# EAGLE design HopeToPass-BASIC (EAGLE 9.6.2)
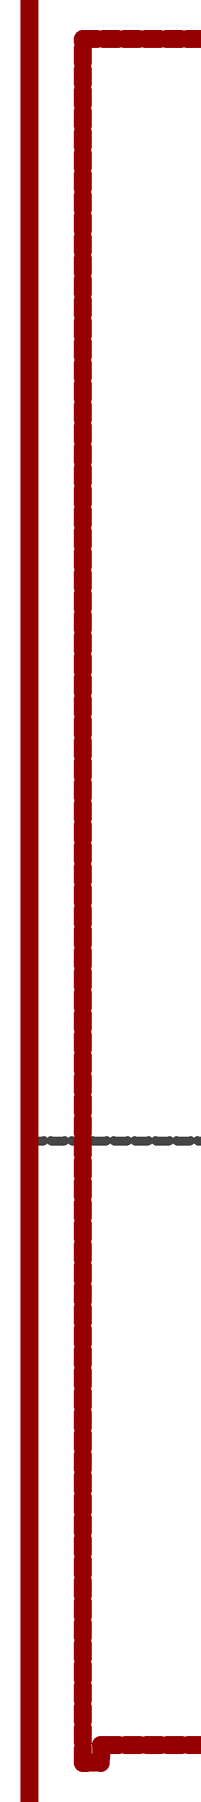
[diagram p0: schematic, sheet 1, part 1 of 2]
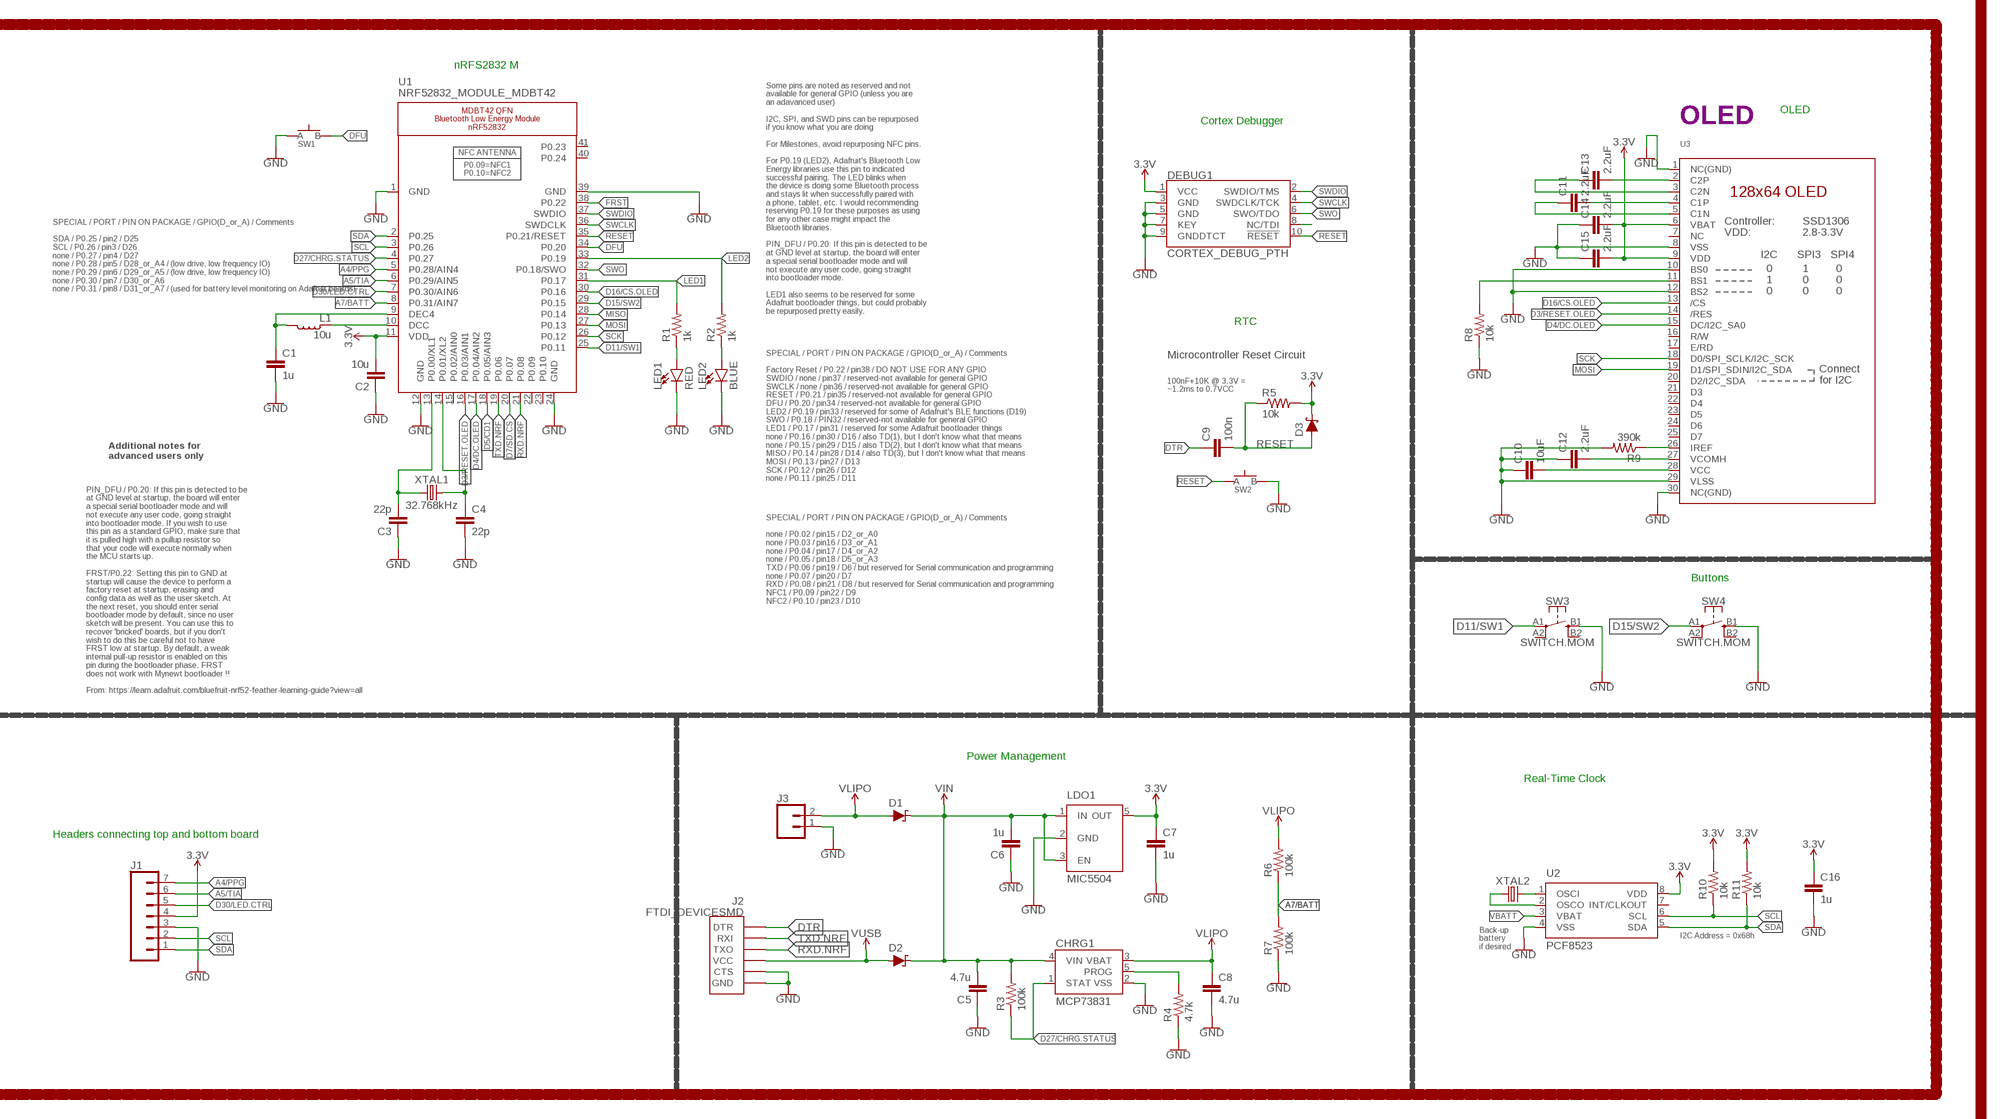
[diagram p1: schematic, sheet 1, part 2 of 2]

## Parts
C1  1u  CAPACITOR0603  [C0603]
C2  10u  CAPACITOR0805  [C0805]
C3  22p  CAPACITOR0603  [C0603]
C4  22p  CAPACITOR0603  [C0603]
C5  4.7u  CAPACITOR0603  [C0603]
C6  1u  CAPACITOR0603  [C0603]
C7  1u  CAPACITOR0603  [C0603]
C8  4.7u  CAPACITOR0603  [C0603]
C9  100n  CAPACITOR0603  [C0603]
C10  10uF  CAPACITOR0603  [C0603]
C11  2.2uF  CAPACITOR0603  [C0603]
C12  2.2uF  CAPACITOR0603  [C0603]
C13  2.2uF  CAPACITOR0603  [C0603]
C14  2.2uF  CAPACITOR0603  [C0603]
C15  2.2uF  CAPACITOR0603  [C0603]
C16  1u  CAPACITOR0603  [C0603]
CHRG1  MCP73831  [SOT23-5]
D1  SCHOTTKY-USC  [USC]
D2  SCHOTTKY-USC  [USC]
D3  SCHOTTKY-USC  [USC]
DEBUG1  CORTEX_DEBUG_PTH  [2X5-PTH-1.27MM]
J1  CONN_07-1.27MM  [1X07_1.27MM]
J2  FTDI_DEVICESMD  [FTDI-SMD]
J3  CONN_02  [1X02]
L1  10u  INDUCTOR0603  [L0603]
LDO1  MIC5504  [SOT23-5]
LED1  RED  LED0603  [LED-0603]
LED2  BLUE  LED0603  [LED-0603]
R1  1k  RESISTOR0603  [R0603]
R2  1k  RESISTOR0603  [R0603]
R3  100k  RESISTOR0603  [R0603]
R4  4.7k  RESISTOR0603  [R0603]
R5  10k  RESISTOR0603  [R0603]
R6  100k  RESISTOR0603  [R0603]
R7  100k  RESISTOR0603  [R0603]
R8  10k  RESISTOR0603  [R0603]
R9  390k  RESISTOR0603  [R0603]
R10  10k  RESISTOR0603  [R0603]
R11  10k  RESISTOR0603  [R0603]
SW1  SPST-PTS830GG140-COPY.1-3  [BUTTON-GULLWING]
SW2  SPST-PTS830GG140-COPY.1-3  [BUTTON-GULLWING]
SW3  SWITCH.MOM  [TACTILE_SWITCH_SMD_6.2MM_TALL]
SW4  SWITCH.MOM  [TACTILE_SWITCH_SMD_6.2MM_TALL]
U1  NRF52832_MODULE_MDBT42  [BLE_MODULE_RAYTAC_MDBT42]
U2  PCF8523  [SO8]
U3  DISP_OLED_UG-2864HSWEG01-NO-WRAPAROUND  [UG-2864HSWEG01_0.96IN_NO-WRAPAROUND]
XTAL1  32.768kHz  CRYSTALECS-.327-12.5-12-C-TR  [2-SMD.NOLEAD.2.0MMTO1.2MM]
XTAL2  32.7680kHz  CRYSTALECS-.327-12.5-12-C-TR  [2-SMD.NOLEAD.2.0MMTO1.2MM]

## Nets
3.3V: C2.2 C7.1 C14.2 C15.2 C16.1 D3.-(C) DEBUG1.1(VCC) J1.4 LDO1.5(OUT) R5.2 R10.2 R11.2 U1.11(VDD) U2.8(VDD) U3.6(VBAT) U3.9(VDD)
A4/PPG: J1.7 U1.5(P0.28/AIN4)
A5/TIA: J1.6 U1.6(P0.29/AIN5)
A7/BATT: R6.1 R7.2 U1.8(P0.31/AIN7)
D3/RESET.OLED: U1.16(P0.03/AIN1) U3.14(/RES)
D4/DC.OLED: U1.17(P0.04/AIN2) U3.15(DC/I2C_SA0)
D5/CD1: U1.18(P0.05/AIN3)
D7/SD.CS: U1.20(P0.07)
D11/SW1: SW3.A1 U1.25(P0.11)
D15/SW2: SW4.A1 U1.29(P0.15)
D16/CS.OLED: U1.30(P0.16) U3.13(/CS)
D27/CHRG.STATUS: CHRG1.1(STAT) R3.1 U1.4(P0.27)
D30/LED.CTRL: J1.5 U1.7(P0.30/AIN6)
DFU: SW1.3(B) U1.34(P0.20)
DTR: C9.1 J2.DTR
FRST: U1.38(P0.22)
GND: C1.2 C2.1 C3.1 C4.2 C5.1 C6.1 C7.2 C8.2 C10.1 C12.1 C14.1 C15.1 C16.2 CHRG1.2(VSS) DEBUG1.3(GND) DEBUG1.5(GND) DEBUG1.7(KEY) DEBUG1.9(GNDDTCT) J1.3 J2.CTS J2.GND J3.1 LDO1.2(GND) LED1.C LED2.C R4.1 R7.1 R8.1 R9.2 SW1.1(A) SW2.3(B) SW3.B1 SW4.B1 U1.1(GND) U1.12(GND) U1.24(GND) U1.39(GND) U2.4(VSS) U3.1(NC(GND)) U3.8(VSS) U3.10(BS0) U3.12(BS2) U3.29(VLSS) U3.30(NC(GND))
LED1: R1.2 U1.31(P0.17)
LED2: R2.2 U1.33(P0.19)
MISO: U1.28(P0.14)
MOSI: U1.27(P0.13) U3.19(D1/SPI_SDIN/I2C_SDA)
N$1: R8.2 U3.11(BS1)
N$2: R9.1 U3.26(IREF)
N$3: C13.2 U3.2(C2P)
N$4: C3.2 U1.13(P0.00/XL1) XTAL1.P$1
N$5: C13.1 U3.3(C2N)
N$6: C4.1 U1.14(P0.01/XL2) XTAL1.P$2
N$7: C11.2 U3.4(C1P)
N$8: C11.1 U3.5(C1N)
N$9: LED1.A R1.1
N$10: LED2.A R2.1
N$11: L1.1 U1.10(DCC)
N$12: C1.1 L1.2 U1.9(DEC4)
N$13: C10.2 U3.28(VCC)
N$14: DEBUG1.8(NC/TDI)
N$15: C12.2 U3.27(VCOMH)
N$17: CHRG1.5(PROG) R4.2
N$21: U2.2(OSCO) XTAL2.P$1
N$22: U2.1(OSCI) XTAL2.P$2
RESET: C9.2 D3.+(A) DEBUG1.10(!RESET) R5.1 SW2.1(A) U1.35(P0.21/RESET)
RXD.NRF: J2.TXO U1.21(P0.08)
SCK: U1.26(P0.12) U3.18(D0/SPI_SCLK/I2C_SCK)
SCL: J1.2 R10.1 U1.3(P0.26) U2.6(SCL)
SDA: J1.1 R11.1 U1.2(P0.25) U2.5(SDA)
SWCLK: DEBUG1.4(SWDCLK/TCK) U1.36(SWDCLK)
SWDIO: DEBUG1.2(SWDIO/TMS) U1.37(SWDIO)
SWO: DEBUG1.6(SWO/TDO) U1.32(P0.18/SWO)
TXD.NRF: J2.RXI U1.19(P0.06)
V_USB: D2.+(A) J2.VCC ; supply symbol labelled VUSB
VBATT: U2.3(VBAT)
VIN: C5.2 C6.2 CHRG1.4(VIN) D1.-(C) D2.-(C) LDO1.1(IN) LDO1.3(EN) R3.2
VLIPO: C8.1 CHRG1.3(VBAT) D1.+(A) J3.2 R6.2
Unconnected: SW3.A2 SW3.B2 SW4.A2 SW4.B2 U1.15(P0.02/AIN0) U1.22(P0.09) U1.23(P0.10) U1.40(P0.24) U1.41(P0.23) U2.7(INT/CLKOUT) U3.7(NC) U3.16(R/W) U3.17(E/RD) U3.20(D2/I2C_SDA) U3.21(D3) U3.22(D4) U3.23(D5) U3.24(D6) U3.25(D7)

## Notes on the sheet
- nRFS2832 M
- OLED
- Cortex Debugger | OLED
- SPECIAL / PORT / PIN ON PACKAGE / GPIO(D_or_A) / Comments
  
  SDA / P0.25 / pin2 / D25
  SCL / P0.26 / pin3 / D26
  none / P0.27 / pin4 / D27
  none / P0.28 / pin5 / D28_or_A4 / (low drive, low frequency IO)
  none / P0.29 / pin6 / D29_or_A5 / (low drive, low frequency IO)
  none / P0.30 / pin7 / D30_or_A6
  none / P0.31 / pin8 / D31_or_A7 / (used for battery level monitoring on Adafruit boards)
- Some pins are noted as reserved and not
  available for general GPIO (unless you are
  an adavanced user)
  
  I2C, SPI, and SWD pins can be repurposed
  if you know what you are doing
  
  For Milestones, avoid repurposing NFC pins.
  
  For P0.19 (LED2), Adafruit's Bluetooth Low
  Energy libraries use this pin to indicated
  successful pairing. The LED blinks when
  the device is doing some Bluetooth process
  and stays lit when successfully paired with
  a phone, tablet, etc. I would recommending
  reserving P0.19 for these purposes as using
  for any other case might impact the
  Bluetooth libraries.
  
  PIN_DFU / P0.20: If this pin is detected to be
  at GND level at startup, the board will enter
  a special serial bootloader mode and will
  not execute any user code, going straight
  into bootloader mode.
  
  LED1 also seems to be reserved for some
  Adafruit bootloader things, but could probably
  be repurposed pretty easily.
- RTC
- Microcontroller Reset Circuit
- 100nF+10K @ 3.3V =
  ~1.2ms to 0.7VCC
- Additional notes for
  advanced users only
- SPECIAL / PORT / PIN ON PACKAGE / GPIO(D_or_A) / Comments
  
  Factory Reset / P0.22 / pin38 / DO NOT USE FOR ANY GPIO
  SWDIO / none / pin37 / reserved-not available for general GPIO
  SWCLK / none / pin36 / reserved-not available for general GPIO
  RESET / P0.21 / pin35 / reserved-not available for general GPIO
  DFU / P0.20 / pin34 / reserved-not available for general GPIO
  LED2 / P0.19 / pin33 / reserved for some of Adafruit's BLE functions (D19)
  SWO / P0.18 / PIN32 / reserved-not available for general GPIO
  LED1 / P0.17 / pin31 / reserved for some Adafruit bootloader things
  none / P0.16 / pin30 / D16 / also TD(1), but I don't know what that means
  none / P0.15 / pin29 / D15 / also TD(2), but I don't know what that means
  MISO / P0.14 / pin28 / D14 / also TD(3), but I don't know what that means
  MOSI / P0.13 / pin27 / D13
  SCK / P0.12 / pin26 / D12
  none / P0.11 / pin25 / D11
- Buttons
- SPECIAL / PORT / PIN ON PACKAGE / GPIO(D_or_A) / Comments
  
  none / P0.02 / pin15 / D2_or_A0
  none / P0.03 / pin16 / D3_or_A1
  none / P0.04 / pin17 / D4_or_A2
  none / P0.05 / pin18 / D5_or_A3
  TXD / P0.06 / pin19 / D6 / but reserved for Serial communication and programming
  none / P0.07 / pin20 / D7
  RXD / P0.08 / pin21 / D8 / but reserved for Serial communication and programming
  NFC1 / P0.09 / pin22 / D9
  NFC2 / P0.10 / pin23 / D10
- PIN_DFU / P0.20: If this pin is detected to be
  at GND level at startup, the board will enter
  a special serial bootloader mode and will
  not execute any user code, going straight
  into bootloader mode. If you wish to use
  this pin as a standard GPIO, make sure that
  it is pulled high with a pullup resistor so
  that your code will execute normally when
  the MCU starts up.
  
  FRST/P0.22: Setting this pin to GND at
  startup will cause the device to perform a
  factory reset at startup, erasing and
  config data as well as the user sketch. At
  the next reset, you should enter serial
  bootloader mode by default, since no user
  sketch will be present. You can use this to
  recover 'bricked' boards, but if you don't
  wish to do this be careful not to have
  FRST low at startup. By default, a weak
  internal pull-up resistor is enabled on this
  pin during the bootloader phase. FRST
  does not work with Mynewt bootloader !!
  
  From: https://learn.adafruit.com/bluefruit-nrf52-feather-learning-guide?view=all
- Power Management
- Real-Time Clock
- Headers connecting top and bottom board
- I2C Address = 0x68h
- Back-up
  battery
  if desired

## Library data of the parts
C1-C16 = LinnesLab-Passives:CAPACITOR
CHRG1 = LinnesLab-Power:MCP73831: MCP73831T Li-Ion, Li-Pol Controller Miniature single cell, fully integrated Li-Ion, Li-polymer charge management controller Datasheet SparkFun Products: SparkFun ESP32 Thing SparkFun 9DoF Razor IMU M0; PROD_ID: IC-09995
D1-D3 = LinnesLab-DiscreteSemi:SCHOTTKY: Schottky diode
DEBUG1 = LinnesLab-Connectors:CORTEX_DEBUG: Cortex Debug Connector - 10 pin Supports JTAG debug, Serial Wire debug, and Serial Wire Viewer. PTH and SMD connector options available. General Connector Information Products: PTH Connector -via Digi-Key SparkFun PSoc SparkFun T
J1 = LinnesLab-Connectors:CONN_07: Multi connection point. Often used as Generic Header-pin footprint for 0.1 inch spaced/style header connections On any of the 0.1 inch spaced packages, you can populate with these: Break Away Headers - Straight (PRT-00116) Break Away Male Headers - Right Angle (PRT-00553) Female Headers (PRT-00115)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
J2 = LinnesLab-Connectors:FTDI_DEVICE
J3 = LinnesLab-Connectors:CONN_02: Multi connection point. Often used as Generic Header-pin footprint for 0.1 inch spaced/style header connections
L1 = LinnesLab-Passives:INDUCTOR
LDO1 = LinnesLab-Power:MIC5504: MIC5504 Voltage Regulator Output Voltages: 1.0V to 3.3V Input Voltages: 2.5V to 5.5V Link to Datasheet http://ww1.microchip.com/downloads/en/DeviceDoc/MIC550X.pdf
LED1 LED2 = LinnesLab-LED:LED: LED (Generic)
R1-R11 = LinnesLab-Passives:RESISTOR
SW1 SW2 = LinnesLab-Switches:SPST-PTS830GG140-COPY
SW3 SW4 = LinnesLab-Switches:SWITCH.MOM: PTS645SM43SMTR92 LFS
U1 = LinnesLab-Microcontrollers:NRF52832_MODULE_MDBT42: MDBT42 - BLE Module (nRF52832 QFN) VDD: 1.7-3.6V
U2 = LinnesLab-Clocks:PCF8523; DIGIKEY: 568-5306-1-ND; I2C_ADDRESS: 0x68h; MFN: PCF8523T/1,118; MFN_MANUFACTURER: NXP USA Inc.
U3 = LinnesLab-Displays:DISP_OLED_UG-2864HSWEG01: UG-2864HSWEG01 OLED display Both 1.3" and 0.96" models share the same FPC tab footprint, only the screen dimensions vary.
XTAL1 XTAL2 = LinnesLab-Clocks:CRYSTAL; DIGIKEY: XC2288CT-ND; FREQ: 32.7680KHZ; LOAD_CAP: 12.5pF

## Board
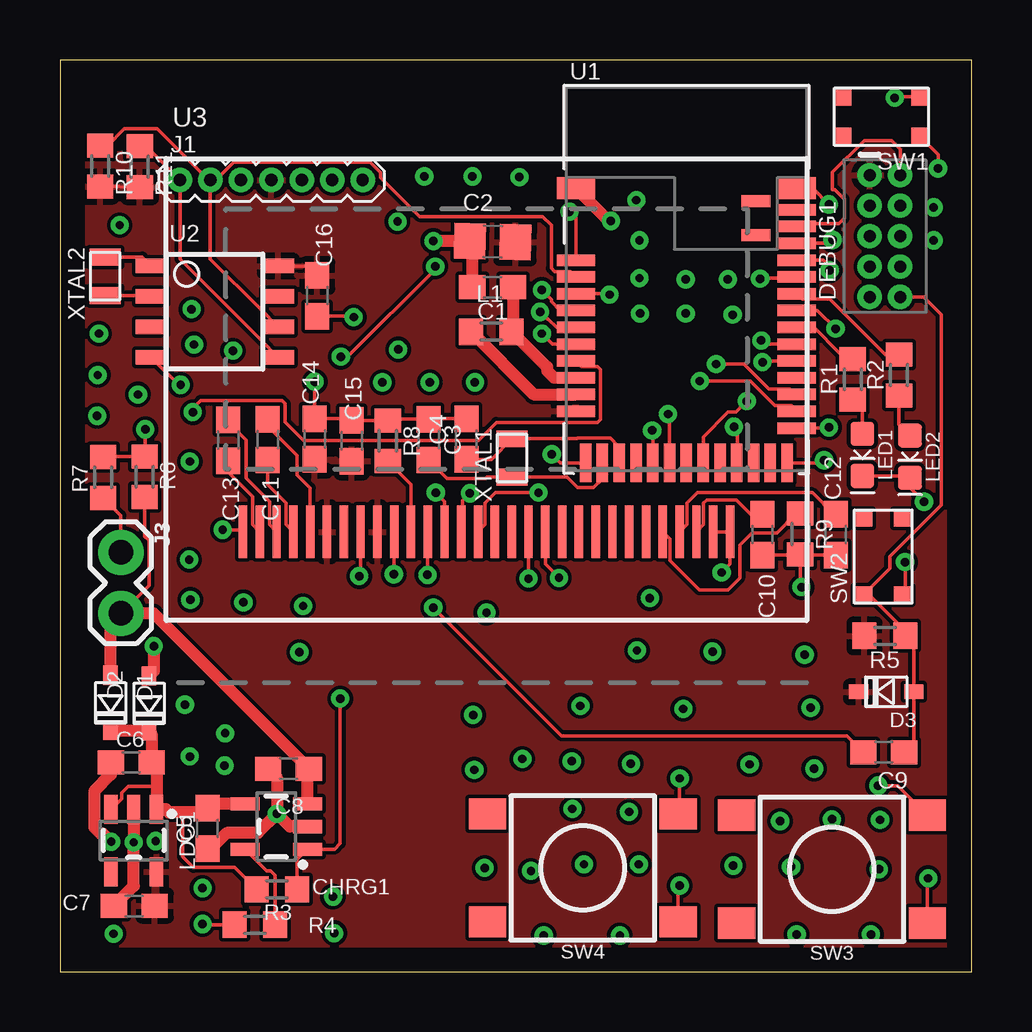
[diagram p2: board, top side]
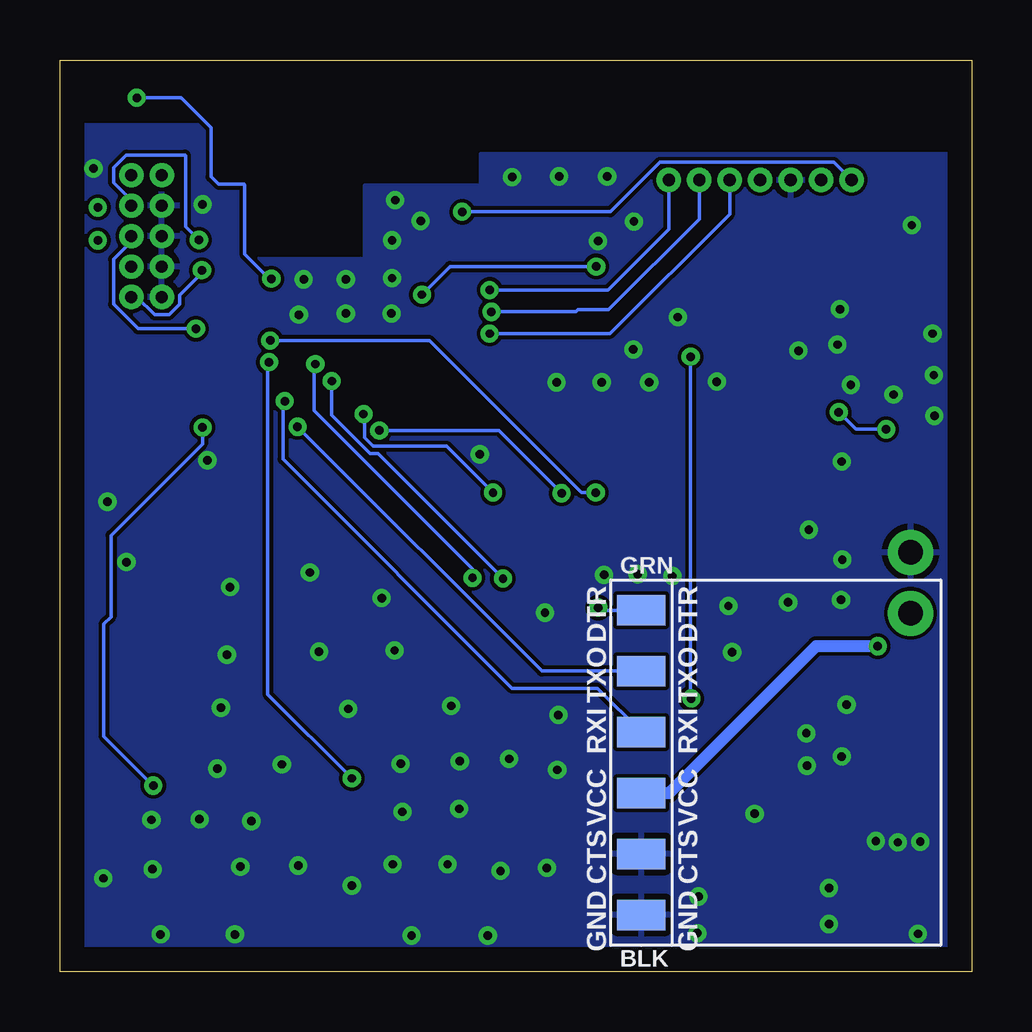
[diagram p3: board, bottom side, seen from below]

Size 38 x 38 mm. Coordinates in mm from the lower left corner, seen from the top.
Outline: 0,0 38,0 38,38 0,38 0,0
Copper layers (1*16): Top 0.035mm / dielectric 1.5mm / Bottom 0.035mm
Design rules "default": minimum track width 6mil, minimum drill 0.35mm, track to track 6mil, track to pad 6mil, pad to pad 6mil, via to via 6mil, smd to smd 6mil, copper to edge 40mil, drill to drill 6mil, minimum pad ring 10mil, minimum via ring 8mil, stop-mask expansion 4mil, vias tented up to drill 0mil, thermal gap 10mil

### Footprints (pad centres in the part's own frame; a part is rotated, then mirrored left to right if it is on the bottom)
C0603 = smd 1.1 x 1: 1 -0.85,0; 2 0.85,0
C0805 = smd 1.3 x 1.5: 1 -0.95,0; 2 0.95,0
SOT23-5 = smd 0.55 x 1.2: 1 -0.95,-1.3; 2 0,-1.3; 3 0.95,-1.3; 4 0.95,1.3; 5 -0.95,1.3
USC = smd 0.8 x 0.6: + -1.15,0; - 1.15,0
2X5-PTH-1.27MM = drill 0.508 pad 1: 1 -2.54,-0.635; 2 -2.54,0.635; 3 -1.27,-0.635; 4 -1.27,0.635; 5 0,-0.635; 6 0,0.635; 7 1.27,-0.635; 8 1.27,0.635; 9 2.54,-0.635; 10 2.54,0.635
1X07_1.27MM = drill 0.508 pad 1: 1 0,0; 2 1.27,0; 3 2.54,0; 4 3.81,0; 5 5.08,0; 6 6.35,0; 7 7.62,0
FTDI-SMD = smd 1.27 x 2.03: CTS 3.81,0; DTR -6.35,0; GND 6.35,0; RXI -1.27,0; TXO -3.81,0; VCC 1.27,0
1X02 = drill 1.016 pad 1.88: 1 0,0; 2 2.54,0
L0603 = smd 1 x 1.1: 1 -0.85,0; 2 0.85,0
LED-0603 = smd 1 x 1: A -0.877,0; C 0.877,0
R0603 = smd 1 x 1.1: 1 -0.85,0; 2 0.85,0
BUTTON-GULLWING = smd 0.7 x 0.75: 1 -1.6,0.825; 2 1.6,0.825; 3 -1.6,-0.825; 4 1.6,-0.825
TACTILE_SWITCH_SMD_6.2MM_TALL = smd 1.55 x 1.3: A1 -3.975,-2.25; A2 3.975,-2.25; B1 -3.975,2.25; B2 3.975,2.25
BLE_MODULE_RAYTAC_MDBT42 = smd 1.6 x 0.9: 1 -4.6,3.8; 39 4.6,3.8 | smd 1.6 x 0.48: 2 -4.6,0.8; 3 -4.6,0.1; 4 -4.6,-0.6; 5 -4.6,-1.3; 6 -4.6,-2; 7 -4.6,-2.7; 8 -4.6,-3.4; 9 -4.6,-4.1; 10 -4.6,-4.8; 11 -4.6,-5.5; 25 4.6,-6.2; 26 4.6,-5.5; 27 4.6,-4.8; 28 4.6,-4.1; 29 4.6,-3.4; 30 4.6,-2.7; 31 4.6,-2; 32 4.6,-1.3; 33 4.6,-0.6; 34 4.6,0.1; 35 4.6,0.8; 36 4.6,1.5; 37 4.6,2.2; 38 4.6,2.9 | smd 0.48 x 1.6: 12 -4.2,-7.65; 13 -3.5,-7.65; 14 -2.8,-7.65; 15 -2.1,-7.65; 16 -1.4,-7.65; 17 -0.7,-7.65; 18 0,-7.65; 19 0.7,-7.65; 20 1.4,-7.65; 21 2.1,-7.65; 22 2.8,-7.65; 23 3.5,-7.65; 24 4.2,-7.65 | smd 1.2 x 0.5: 40 2.9,3.25; 41 2.9,1.85
SO8 = smd 1.3 x 0.6: 1 -2.65,1.905; 2 -2.65,0.635; 3 -2.65,-0.635; 4 -2.65,-1.905; 5 2.65,-1.905; 6 2.65,-0.635; 7 2.65,0.635; 8 2.65,1.905
UG-2864HSWEG01_0.96IN_NO-WRAPAROUND = smd 0.35 x 2.2: 1 -10.15,-1.2; 2 -9.45,-1.2; 3 -8.75,-1.2; 4 -8.05,-1.2; 5 -7.35,-1.2; 6 -6.65,-1.2; 7 -5.95,-1.2; 8 -5.25,-1.2; 9 -4.55,-1.2; 10 -3.85,-1.2; 11 -3.15,-1.2; 12 -2.45,-1.2; 13 -1.75,-1.2; 14 -1.05,-1.2; 15 -0.35,-1.2; 16 0.35,-1.2; 17 1.05,-1.2; 18 1.75,-1.2; 19 2.45,-1.2; 20 3.15,-1.2; 21 3.85,-1.2; 22 4.55,-1.2; 23 5.25,-1.2; 24 5.95,-1.2; 25 6.65,-1.2; 26 7.35,-1.2; 27 8.05,-1.2; 28 8.75,-1.2; 29 9.45,-1.2; 30 10.15,-1.2
2-SMD.NOLEAD.2.0MMTO1.2MM = smd 0.7 x 1.3: P$1 -0.8,0; P$2 0.8,0

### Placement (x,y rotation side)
C1  18.03,28.52 180 top
C2  18.03,30.43 358.7 top
C3  15.37,22.17 270 top
C4  16.94,22.2 90 top
C5  6.15,5.97 90 top
C6  2.97,8.71 0 top
C7  3.1,2.74 180 top
C8  9.53,8.46 180 top
C9  34.34,9.14 0 top
C10  29.29,18.21 90 top
C11  8.66,22.17 270 top
C12  32.33,18.21 90 top
C13  7.01,22.15 270 top
C14  10.62,22.2 270 top
C15  12.17,22.12 270 top
C16  10.72,28.17 270 top
CHRG1  9.02,6.05 90 top
D1  2.11,11.2 270 top
D2  3.71,11.18 270 top
D3  34.44,11.66 180 top
DEBUG1  34.39,30.66 270 top
J1  5,33 0 top
J2  13.77,8.71 270 bottom
J3  2.54,17.48 270 top
L1  17.98,26.67 0 top
LDO1  3.07,5.46 180 top
LED1  33.45,21.54 270 top
LED2  35.43,21.46 270 top
R1  33.05,24.69 90 top
R2  34.98,24.87 90 top
R3  9.04,3.43 180 top
R4  8.13,1.96 0 top
R5  34.39,14 180 top
R6  3.53,20.62 270 top
R7  1.8,20.6 90 top
R8  13.67,22.12 270 top
R9  30.86,18.24 270 top
R10  1.68,33.58 270 top
R11  3.33,33.55 270 top
SW1  34.24,35.64 180 top
SW2  34.32,17.3 90 top
SW3  32.18,4.27 180 top
SW4  21.79,4.32 180 top
U1  26.11,28.85 0 top
U2  6.45,27.51 0 top
U3  17.78,19.53 0 top
XTAL1  18.85,21.41 90 top
XTAL2  1.88,28.98 90 top

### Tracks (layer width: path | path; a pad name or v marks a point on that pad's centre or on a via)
3.3V
  Top 0.152: R11.2 1.68,32.75 R10.2 | U2.8 10.32,29.41 C16.1
  pour Top: 0.56,34.14 20.47,34.14 20.47,32.84 25.32,32.84 25.32,29.74 30.15,29.74 30.15,32.84 31.78,32.84 31.78,32.97 31.78,35.31 37.77,35.31 37.77,0.41 0.56,0.41
A4/PPG  (via drill 0.35)
  Top 0.152: v20.09,28.41 20.48,28.02 20.48,27.92 20.85,27.55 U1.5
  Bottom 0.152: J1.7 12.62,30.94 15.15,28.41 v20.09,28.41
A5/TIA  (via drill 0.35)
  Top 0.152: U1.6 20.69,26.85 20.34,27.2 20.32,27.2 v20.02,27.5
  Bottom 0.152: v20.02,27.5 16.49,27.5 16.41,27.58 15.14,27.58 11.35,31.37 J1.6
A7/BATT  (via drill 0.35)
  Top 0.152: R7.2 1.83,21.48 R6.1 3.56,21.5 v3.56,22.61 | U1.8 21.74,25.22 22.41,25.22 22.54,25.09 22.54,23.02 22.41,22.89 18.2,22.89 17.45,22.14 10.16,22.14 9.39,22.9 9.39,23.67 9.26,23.8 5.86,23.8 5.54,23.48 v5.54,23.32
  Bottom 0.152: v5.54,23.32 4.83,22.61 v3.56,22.61
D3/RESET.OLED  (via drill 0.35)
  Top 0.152: U3.14 16.78,18.39 16.78,19.63 v17.09,19.94 | v24.69,22.55 24.71,22.53 U1.16
  Bottom 0.152: v17.09,19.94 19.7,22.55 v24.69,22.55
D4/DC.OLED  (via drill 0.35)
  Top 0.152: U1.17 25.41,23.18 v25.35,23.24 | U3.15 17.73,18.63 17.73,19.53 18.16,19.96 v19.95,19.96
  Bottom 0.152: v19.95,19.96 21.88,21.9 24.94,21.9 25.3,22.25 25.3,23.19 v25.35,23.24
D11/SW1  (via drill 0.35)
  Top 0.152: U1.25 32.03,22.65 v32.05,22.68 | SW3.A1 34.93,7.75 v34.11,7.75
  Bottom 0.152: v32.05,22.68 32.05,22 35.87,18.18 35.87,14.79 36.17,14.48 36.17,9.8 v34.11,7.75
D15/SW2  (via drill 0.35)
  Top 0.152: U1.29 29.34,25.45 v29.29,25.4 | v25.83,8.05 25.83,6.63 SW4.A1
  Bottom 0.152: v29.29,25.4 29.34,25.35 29.34,11.56 v25.83,8.05
D16/CS.OLED  (via drill 0.35)
  Top 0.152: U3.13 16.03,19.6 v15.67,19.96 | v29.23,26.31 29.39,26.15 U1.30
  Bottom 0.152: v15.67,19.96 16.25,19.96 22.6,26.31 v29.23,26.31
D27/CHRG.STATUS  (via drill 0.35)
  Top 0.152: R3.1 9.89,4.67 CHRG1.1 11.45,5.09 11.68,5.33 v11.68,11.38 | U1.4 22.88,28.25 v22.91,28.22 | v15.65,29.39 15.65,29.29 11.99,25.63 v11.71,25.63
  Bottom 0.152: v22.91,28.22 21.74,29.39 v15.65,29.39 | v11.71,25.63 11.71,11.4 v11.68,11.38
D30/LED.CTRL  (via drill 0.35)
  Top 0.152: U1.7 20.53,26.15 v20.09,26.59
  Bottom 0.152: v20.09,26.59 15.06,26.59 10.08,31.58 J1.5
DFU  (via drill 0.35)
  Top 0.152: SW1.3 34.84,36.46 v34.8,36.42 | v29.18,28.88 29.21,28.91 30.66,28.91 U1.34
  Bottom 0.152: v29.18,28.88 29.28,28.88 30.3,29.9 30.3,32.79 30.33,32.82 31.38,32.82 31.7,33.13 31.7,35.18 32.94,36.42 v34.8,36.42
DTR  (via drill 0.35)
  Top 0.152: C9.1 32.8,9.83 20.9,9.83 v15.56,15.17
  Bottom 0.152: v15.56,15.17 15.45,15.06 J2.DTR
GND  (via drill 0.35)
  Top 0.152: LED1.C 35.36,20.66 LED2.C 35.43,20.17 v36.02,19.58 | SW1.1 36.61,34.05 v36.61,33.48 | SW2.3 35.23,15.79 v35.23,17.07 | SW3.B1 36.16,3.85 v36.2,3.89 | SW4.B1 25.77,3.52 v25.83,3.58 | U3.1 7.55,18.41 v6.78,18.41 | U3.8 12.53,16.54 v12.47,16.48 | U3.10 13.93,16.57 v13.92,16.56 | U3.12 v15.33,16.55 v15.32,16.54 | v10.62,24.59 C14.1 12.09,23.05 C15.1 R8.1 13.72,23.02 C3.1 15.39,23.05 C4.2 | U1.12 20.86,21.2 v20.5,21.57 | R4.1 5.97,1.96 v5.94,1.98 | J3.1 2.54,19.01 R7.1 | C10.1 30.84,17.36 | 30.84,17.36 R9.2 30.86,16.08 v30.91,16.03 | U3.29 U3.30 27.93,16.98 v27.58,16.64 | C12.1 30.84,17.36 | U1.24 31.75,21.2 v31.85,21.31 | U1.39 31.38,32.65 v32.05,31.98 | U2.4 4.95,24.46 v5.03,24.46 | C16.2 12.2,27.32 v12.24,27.28
  Top 0.508: 2.12,8.62 C6.1 2.12,8.21 1.44,7.53 1.44,5.99 1.68,5.75 1.79,5.75 v2.13,5.41 | LDO1.2 v3.07,5.38 3.07,3.57 C7.2 | CHRG1.2 9.58,6.04 v9.04,6.58 | v9.04,6.58 8.24,5.78 6.95,5.78 6.29,5.12 C5.1 | C8.2 9.04,8.09 v9.04,6.58 | U1.1 22.87,31.29 v22.96,31.29 | C1.2 17.18,30.35 C2.1 v15.57,30.45
  other vias: 2.24,1.57 3.99,5.44 31.45,8.46 33.81,1.55 30.71,1.55 23.8,8.66 23.34,1.5 20.17,1.5 19.28,8.86 11.43,1.6 11.38,3.12 5.94,3.48 5.41,8.97 6.88,9.93 5.21,11.13 5.38,17.17 5.41,21.26 15.42,24.56 14.07,31.27 17.7,4.32 19.63,4.19 21.84,4.47 34.14,4.27 30.48,4.37 1.57,24.87 1.63,26.59 17.22,10.69 24.05,13.39 27.2,13.34 31.04,13.21 6.86,8.59 19.15,33.12 17.2,33.15 15.19,33.15 7.21,25.88 5.59,26.14 5.49,27.61 14.1,25.93 10.13,15.24 5.44,15.49 2.49,31.11 24.16,30.48 24.03,32.16 24.18,27.43 26.09,27.43 27.84,28.85 28.04,27.38 24.59,15.57 25.98,10.95 21.36,6.78 28.07,4.42 13.44,24.56 1.55,23.16 3.25,24.05 24.16,28.91 26.09,28.85 31.29,11 21.69,11.07 17.27,8.41 21.34,8.76 23.72,6.65 24.13,4.47 28.75,8.64 30.02,6.27 32.18,6.35 34.19,6.32 7.65,15.39 9.98,13.31 17.3,24.56 17.78,14.96
  pour Bottom: 0.48,34.09 20.47,34.09 20.47,32.79 25.3,32.79 25.3,29.72 30.28,29.72 30.28,32.77 31.8,32.77 31.8,35.31 37.67,35.31 37.67,0.43 0.43,0.43
LED1
  Top 0.152: U1.31 31.42,26.85 32.49,25.78 32.8,25.78 R1.2
LED2
  Top 0.152: R2.2 34.41,25.72 32.1,28.03 30.94,28.03 U1.33
MOSI  (via drill 0.35)
  Top 0.152: U3.19 20.23,16.98 v20.8,16.41 | U1.27 30.68,24.03 30.43,24.29 29.54,24.29 28.5,25.32 v27.36,25.32
  Bottom 0.152: v20.8,16.41 20.8,16.79 27.41,23.39 27.41,25.27 v27.36,25.32
N$1
  Top 0.152: R8.2 14.63,20.31 U3.11
N$2
  Top 0.152: R9.1 30.68,19.09 29.88,18.28 28.83,18.28 28.33,17.78 28.33,16.4 27.84,15.91 26.65,15.91 25.43,17.14 25.43,18.04 U3.26
N$3
  Top 0.152: U3.2 8.03,18.63 8.03,19.79 7.01,20.82 C13.2
N$4
  Top 0.152: C3.2 16.15,20.55 17.74,20.55 17.81,20.61 XTAL1.P$1 21.14,20.61 21.58,20.18 22.25,20.18 22.61,20.54 U1.13
N$5
  Top 0.152: U3.3 8.73,18.63 8.73,19.6 7.76,20.57 7.76,22.15 7.01,22.9 C13.1
N$6
  Top 0.152: C4.1 17.98,21.35 XTAL1.P$2 21.56,22.21 21.58,22.23 22.95,22.23 23.31,21.87 U1.14
N$7
  Top 0.152: U3.4 9.43,18.63 9.43,19.53 8.66,20.3 C11.2
N$8
  Top 0.152: U3.5 10.43,20.16 9.89,20.7 9.89,21.52 8.66,22.75 C11.1
N$9
  Top 0.152: R1.1 33.45,23.43 LED1.A
N$10
  Top 0.152: LED2.A 34.98,22.8 R2.1
N$11
  Top 0.508: L1.1 19.75,24.05 U1.10
N$12
  Top 0.508: C1.1 18.88,26.72 L1.2 20.3,25.2 20.3,25.05 20.6,24.75 U1.9
N$13
  Top 0.152: U3.28 26.83,18.63 26.83,19.53 26.96,19.66 28.2,19.66 28.8,19.06 C10.2
N$15
  Top 0.152: U3.27 26.13,18.63 26.13,19.53 26.57,19.97 31.36,19.97 32.26,19.06 C12.2
N$17
  Top 0.152: CHRG1.5 8.6,4.21 8.79,4.21 8.98,4.02 R4.2
N$21
  Top 0.152: XTAL2.P$1 3.76,28.18 U2.2
N$22
  Top 0.152: XTAL2.P$2 3.43,29.78 U2.1
N$25  (via drill 0.35)
  other vias: 36.42,31.85
N$26  (via drill 0.35)
  other vias: 36.42,30.48
RESET  (via drill 0.35)
  Top 0.152: U1.35 31.81,29.65 32.08,29.39 v32.08,29.23 | C9.2 35.59,9.55 D3.+ 35.59,13.64 R5.1 35.24,14.2 33.69,15.76 33.56,15.63 SW2.1 34.6,16.8 34.6,17.3 36.74,19.44 36.74,27.38 36.01,28.12 DEBUG1.10
  Bottom 0.152: DEBUG1.10 34.8,28.12 34.06,27.38 33.45,27.38 33.02,27.81 33.02,28.19 32.08,29.13 v32.08,29.23
RXD.NRF  (via drill 0.35)
  Top 0.152: U1.21 28.25,21.24 28.25,22.56 v28.1,22.71
  Bottom 0.152: v28.1,22.71 17.91,12.52 J2.TXO
SCK  (via drill 0.35)
  Top 0.152: U3.18 v19.53,16.38 | v26.67,24.61 28.78,24.61 29.81,23.59 30.48,23.59 U1.26
  Bottom 0.152: v19.53,16.38 24.74,21.59 25.07,21.59 26.67,23.2 v26.67,24.61
SCL
  Top 0.152: U2.6 8.36,27.61 6.27,29.7 6.27,32.92 | 6.27,32.92 J1.2 6.5,33 7.24,33.74 12.93,33.74 13.36,33.3 13.36,33.1 14.99,31.47 20.12,31.47 20.48,31.11 20.48,29.32 20.62,29.19 21.28,29.19 U1.3 | R10.1 1.98,34.43 2.68,35.13 4.06,35.13 6.27,32.92
SDA  (via drill 0.35)
  Top 0.152: U2.5 8.36,26.34 5,29.7 J1.1 3.6,34.4 R11.1 | v21.23,31.67 21.51,31.4 U1.2
  Bottom 0.152: v21.23,31.67 15.06,31.67 13,33.74 5.74,33.74 J1.1
SWCLK  (via drill 0.35)
  Top 0.152: U1.36 32.06,30.35 v32.21,30.5
  Bottom 0.152: v32.21,30.5 32.77,31.06 32.77,34.01 32.79,34.04 35.23,34.04 35.76,33.5 35.76,32.89 35.03,32.16 DEBUG1.4
SWDIO
  Top 0.152: U1.37 30.84,31.18 32.47,31.18 32.69,31.41 32.69,32.2 32.31,32.59 32.21,32.59 32.21,33.33 33.53,34.65 34.67,34.65 35.03,34.29 DEBUG1.2
SWO  (via drill 0.35)
  Top 0.152: U1.32 31.58,27.55 v32.33,26.8
  Bottom 0.152: DEBUG1.6 35.03,30.43 35.76,29.69 35.76,27.81 34.75,26.8 v32.33,26.8
TXD.NRF  (via drill 0.35)
  Top 0.152: U1.19 26.82,21.22 26.82,22.29 27.85,23.31 28.17,23.31 v28.63,23.77
  Bottom 0.152: J2.RXI 15.6,11.81 19.15,11.81 28.7,21.36 28.7,23.7 v28.63,23.77
V_USB  (via drill 0.35)
  Top 0.508: v3.91,13.56 3.91,12.53 D2.+
  Bottom 0.508: J2.VCC 12.6,7.44 6.48,13.56 v3.91,13.56
VIN
  Top 0.152: LDO1.3 2.57,7.21 2.57,7.46 2.84,7.72 4.02,7.72 | 5.11,6.63 5.11,4.79 5.55,4.34 7.28,4.34 R3.2
  Top 0.508: D1.- 2.13,10.03 D2.- 3.82,9.91 C6.2 4.02,8.51 4.02,7.72 LDO1.1 4.42,6.76 4.55,6.63 5.11,6.63 5.96,6.63 C5.2 6.32,7 CHRG1.4
VLIPO
  Top 0.152: R6.2 3.53,18.14 3.71,17.96 3.71,16.1 J3.2
  Top 0.508: D1.+ 2.11,14.5 J3.2 3.9,14.94 C8.1 10.32,8.4 CHRG1.3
